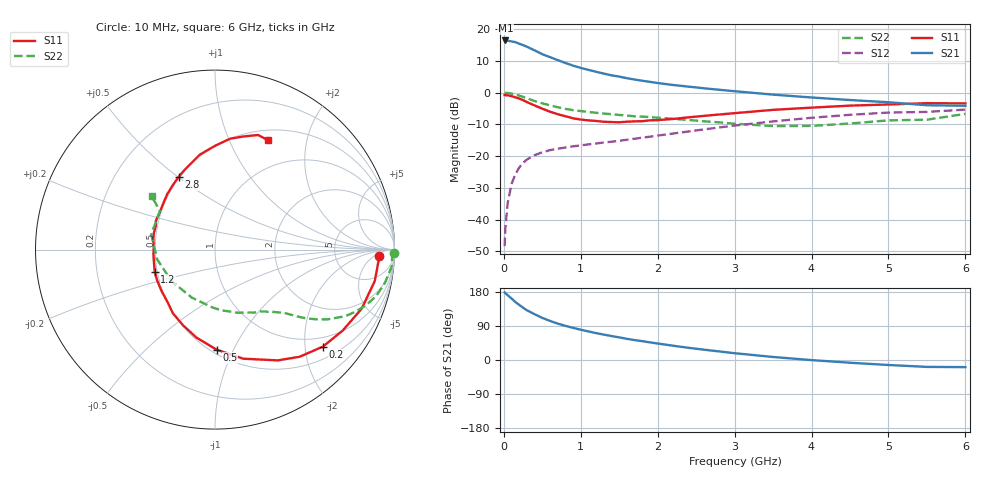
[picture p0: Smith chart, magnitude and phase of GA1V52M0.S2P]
! Infineon Technologies  Discrete & RF Semiconductors
! BF775
! Si NPN RF Bipolar Junction Transistor in SOT23
! VCE = 1.5 V  IC = 2 mA
! Common Emitter S-Parameters:  May  1996
# GHz  S  MA  R  50
!  f  S11  S21  S12  S22
! GHz  MAG  ANG  MAG  ANG  MAG  ANG  MAG  ANG
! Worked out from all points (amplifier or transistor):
!   36 points, 10 MHz to 6 GHz, reference 50 ohm
!   highest |S21| = 16.5 dB at 20 MHz (marker M1)
!   |S21| within 3 dB of that: start of sweep to 388.8 MHz
!   unconditionally stable (mu >= 1): 1.123 GHz to end of sweep
!   at 250 MHz: K = 0.29, MSG = 18.6 dB, |S12| = -22.1 dB
!   at 1.4 GHz: K = 1.13, MAG = 8.3 dB, |S12| = -15.5 dB
!   at 6 GHz: K = 1.04, MAG = -0.6 dB, |S12| = -5.3 dB
!   S11 on the Smith chart (normalised r, x): 10 MHz: 19, -8; 200 MHz: 0.77, -2.39; 500 MHz: 0.53, -0.87; 1.2 GHz: 0.48, -0.14; 2.8 GHz: 0.49, +0.50; 6 GHz: 0.62, +1.40
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0.01  0.9152 -2.3  6.543 178.5  0.0038 86.9  0.9968 -1.0
0.02  0.9125 -4.4  6.65 176.3  0.0073 87.7  0.9883 -2.2
0.05  0.9074 -11.1  6.589 171.0  0.0182 82.7  0.9883 -5.6
0.1  0.8811 -21.9  6.412 162.4  0.0362 76.8  0.966 -10.8
0.15  0.8425 -32.4  6.253 153.0  0.0519 70.9  0.9354 -16.0
0.2  0.8082 -42.0  5.909 145.5  0.066 66.2  0.8986 -20.0
0.25  0.7607 -51.7  5.603 138.1  0.0782 61.4  0.8579 -23.7
0.3  0.7099 -60.4  5.303 131.2  0.0882 57.7  0.8162 -27.0
0.4  0.6278 -75.5  4.638 120.8  0.1034 51.4  0.7393 -31.7
0.5  0.5585 -88.9  4.033 111.1  0.1148 47.3  0.6783 -34.9
0.6  0.5011 -101.9  3.629 103.1  0.1241 44.2  0.63 -37.3
0.7  0.4577 -112.9  3.264 96.1  0.1306 42.5  0.5886 -39.2
0.8  0.425 -123.6  2.935 90.1  0.1364 41.1  0.5551 -40.7
1.1  0.3654 -151.8  2.284 75.3  0.153 40.0  0.4956 -44.9
1.2  0.3579 -160.0  2.132 70.9  0.1578 39.9  0.4811 -46.3
1.6  0.3482 170.3  1.689 55.8  0.181 41.5  0.4347 -52.5
2.2  0.3846 139.0  1.321 37.7  0.2267 42.2  0.3863 -65.4
2.8  0.4523 116.7  1.11 22.6  0.2824 39.7  0.3403 -84.0
3.5  0.5356 99.1  0.931 8.0  0.3521 33.6  0.2972 -115.6
4.5  0.6244 82.1  0.765 -7.2  0.4477 21.3  0.3264 -170.3
5.5  0.6822 69.4  0.633 -18.2  0.4972 6.3  0.3747 144.9
6  0.6768 64.2  0.621 -18.8  0.5407 2.2  0.4623 139.9
